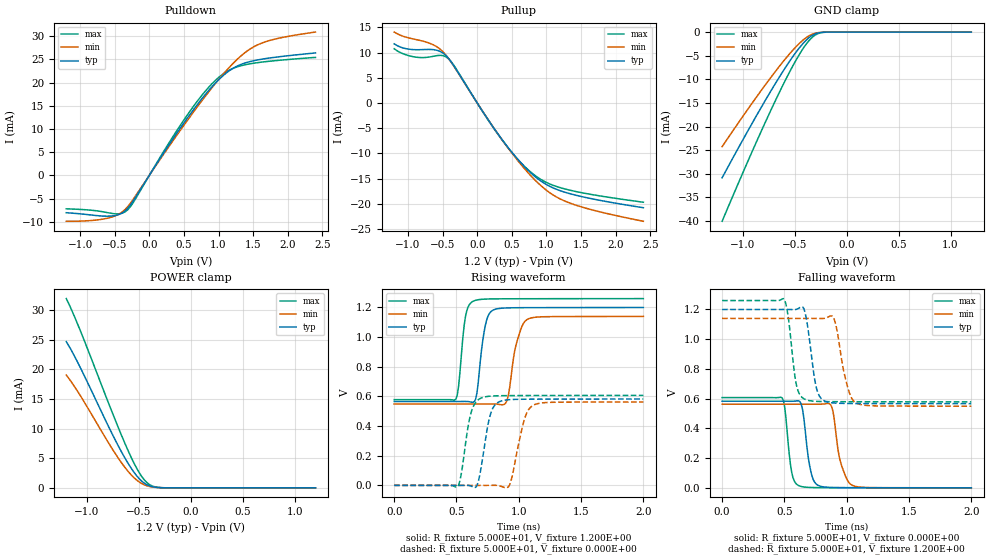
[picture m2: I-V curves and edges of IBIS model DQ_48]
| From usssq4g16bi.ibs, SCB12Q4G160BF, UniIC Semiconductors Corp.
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|   Model DQ_48
[Model] DQ_48
Model_type I/O
Polarity   Non-Inverting
Enable   Active-High
Vinl =  8.300E-01
Vinh =  9.700E-01
Vmeas =  8.400E-01
Rref =  5.000E+01
Vref =  1.200E+00
C_comp   7.774E-13   7.688E-13   7.898E-13
C_comp_pullup   2.832E-13   2.824E-13   2.873E-13
C_comp_pulldown   4.942E-13   4.864E-13   5.024E-13
[Model Spec]
Vinh   9.700E-01   9.250E-01   1.015E+00
Vinl   8.300E-01   7.850E-01   8.750E-01
Vmeas   8.400E-01   7.980E-01   8.820E-01
Vref   1.200E+00   1.140E+00   1.260E+00
Rref   5.000E+01   5.000E+01   5.000E+01
[Temperature Range]   45.000   95.000   -40.000
[Voltage Range]   1.200E+00   1.140E+00   1.260E+00
[C Comp Corner]
C_comp_pullup   2.832E-13   2.824E-13   2.873E-13
C_comp_pulldown   4.942E-13   4.864E-13   5.024E-13
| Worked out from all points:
|   slope of the pulldown table from 0 to 0.18 V, typ, clamps not added: 42.8 ohm
|   slope of the pullup table from 0 to 0.18 V, typ, clamps not added: 47.7 ohm
|   GND clamp passes 1 mA (typ) near -0.35 V on its own axis
|   POWER clamp passes 1 mA (typ) near -0.46 V on its own axis
|   rising waveform, R_fixture 5.000E+01, V_fixture 1.200E+00: 20-80 % time 55.8ps typ, 75.9ps min, 47.2ps max; typ from 0.566 V to 1.2 V
|   rising waveform, R_fixture 5.000E+01, V_fixture 0.000E+00: 20-80 % time 71.2ps typ, 87.3ps min, 68.8ps max; typ from 0 V to 0.583 V
|   falling waveform, R_fixture 5.000E+01, V_fixture 0.000E+00: 20-80 % time 54.1ps typ, 73.3ps min, 45.2ps max; typ from 0.583 V to 0 V
|   falling waveform, R_fixture 5.000E+01, V_fixture 1.200E+00: 20-80 % time 62.7ps typ, 80.9ps min, 56.6ps max; typ from 1.2 V to 0.566 V
[Pulldown]
|Voltage   I(typ)   I(min)   I(max)
-1.2V     -8.065mA   -9.905mA   -7.219mA
-608mV    -8.815mA   -9.258mA   -8.034mA
-423mV    -8.347mA   -8.211mA   -8.276mA
-312mV    -7.111mA   -6.747mA   -7.423mA
-201mV    -4.773mA   -4.47mA    -5.101mA
317mV     7.313mA    6.93mA     7.774mA
613mV     13.65mA    13.14mA    14.36mA
909mV     19.16mA    18.95mA    19.8mA
1.131V    22.28mA    22.87mA    22.48mA
1.39V     24.25mA    26.54mA    23.85mA
1.612V    25mA       28.43mA    24.38mA
2.4V      26.38mA    30.88mA    25.4mA
[Pullup]
|Voltage   I(typ)   I(min)   I(max)
-1.2V     11.73mA    14.08mA    10.77mA
-930mV    10.6mA     12.72mA    9.204mA
-634mV    10.59mA    11.54mA    9.273mA
-523mV    10.14mA    10.52mA    9.452mA
-412mV    8.795mA    8.783mA    8.742mA
180mV     -3.772mA   -3.753mA   -3.834mA
439mV     -8.709mA   -8.796mA   -8.766mA
735mV     -13.35mA   -13.83mA   -13.24mA
994mV     -16.12mA   -17.24mA   -15.71mA
1.179V    -17.29mA   -18.88mA   -16.7mA
1.438V    -18.32mA   -20.31mA   -17.58mA
2.4V      -20.76mA   -23.45mA   -19.67mA
[GND_clamp]
|Voltage   I(typ)   I(min)   I(max)
-1.2V     -30.84mA   -24.25mA   -40.04mA
-875mV    -17.92mA   -13.94mA   -23.52mA
-750mV    -13.19mA   -10.17mA   -17.47mA
-625mV    -8.699mA   -6.602mA   -11.7mA
-525mV    -5.384mA   -3.989mA   -7.412mA
-450mV    -3.179mA   -2.281mA   -4.518mA
-375mV    -1.408mA   -958.6uA   -2.123mA
-325mV    -614.2uA   -404.9uA   -980.6uA
-250mV    -97.6uA    -67.88uA   -160.7uA
-175mV    -8.82uA    -7.635uA   -12.18uA
1.2V      0A         0A         0A
[POWER_clamp]
|Voltage   I(typ)   I(min)   I(max)
-1.2V     24.65mA    19.01mA    31.9mA
-1.15V    23.15mA    17.82mA    30.04mA
-1.075V   20.62mA    15.83mA    26.93mA
-775mV    9.691mA    7.064mA    13.48mA
-625mV    4.722mA    3.212mA    7.078mA
-550mV    2.672mA    1.744mA    4.238mA
-500mV    1.586mA    1.017mA    2.629mA
-450mV    802uA      518.6uA    1.374mA
-400mV    337uA      230.9uA    568.8uA
-350mV    119.1uA    91.13uA    183.1uA
-250mV    9.454uA    10.16uA    10.01uA
1.2V      0A         0A         2.743nA
[Ramp]
| variable   typ   min   max
dV/dt_r   3.495E-01/7.210E-11   3.374E-01/8.826E-11   3.642E-01/6.911E-11
dV/dt_f   3.802E-01/6.338E-11   3.543E-01/8.076E-11   4.089E-01/5.712E-11
R_load = 5.000E+01
[Rising Waveform]
R_fixture= 5.000E+01
V_fixture= 1.200E+00
V_fixture_min= 1.140E+00
V_fixture_max= 1.260E+00
|time   V(typ)   V(min)   V(max)
0s        565.9mV    548.9mV    578.3mV
496ps     565.8mV    548.9mV    583.8mV
572ps     566.1mV    548.9mV    1.138V
643ps     565.4mV    548.9mV    1.245V
731ps     1.077V     549mV      1.256V
790ps     1.18V      549.1mV    1.258V
906ps     1.197V     575.2mV    1.258V
977ps     1.198V     943.9mV    1.259V
1.067ns   1.199V     1.119V     1.259V
2ns       1.2V       1.139V     1.26V
[Rising Waveform]
R_fixture= 5.000E+01
V_fixture= 0.000E+00
V_fixture_min= 0.000E+00
V_fixture_max= 0.000E+00
|time   V(typ)   V(min)   V(max)
0s        386.7nV    981.7nV    169nV
507ps     -153.4uV   1.317uV    -11.54mV
612ps     -3.088mV   11.31uV    474.8mV
664ps     -1.335mV   -52.35uV   569.3mV
708ps     174.2mV    -91.2uV    592.4mV
790ps     517.8mV    447.7uV    603.1mV
918ps     577.6mV    -8.708mV   605.4mV
1.049ns   581.1mV    455.4mV    605.9mV
1.122ns   581.4mV    542.8mV    606mV
2ns       582.5mV    562.4mV    606.9mV
[Falling Waveform]
R_fixture= 5.000E+01
V_fixture= 0.000E+00
V_fixture_min= 0.000E+00
V_fixture_max= 0.000E+00
|time   V(typ)   V(min)   V(max)
0s        583mV      563mV      607.3mV
482ps     583mV      563mV      604.6mV
559ps     582.6mV    563mV      103.9mV
624ps     579.7mV    563mV      12.15mV
712ps     110.6mV    562.9mV    2.691mV
772ps     16.5mV     562.8mV    1.724mV
880ps     2.629mV    544.4mV    1.254mV
949ps     1.617mV    177.9mV    1.118mV
1.04ns    1.24mV     19.66mV    977.6uV
2ns       347.2uV    511uV      257.7uV
[Falling Waveform]
R_fixture= 5.000E+01
V_fixture= 1.200E+00
V_fixture_min= 1.140E+00
V_fixture_max= 1.260E+00
|time   V(typ)   V(min)   V(max)
0s        1.2V       1.14V      1.26V
502ps     1.2V       1.14V      1.264V
598ps     1.201V     1.14V      686.6mV
666ps     1.179V     1.14V      595.4mV
752ps     689.2mV    1.14V      582.3mV
821ps     585.2mV    1.14V      580.5mV
900ps     570.9mV    1.133V     579.9mV
1ns       567.9mV    701.5mV    579.6mV
1.071ns   567.4mV    574.2mV    579.4mV
2ns       566.3mV    549.5mV    578.6mV
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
